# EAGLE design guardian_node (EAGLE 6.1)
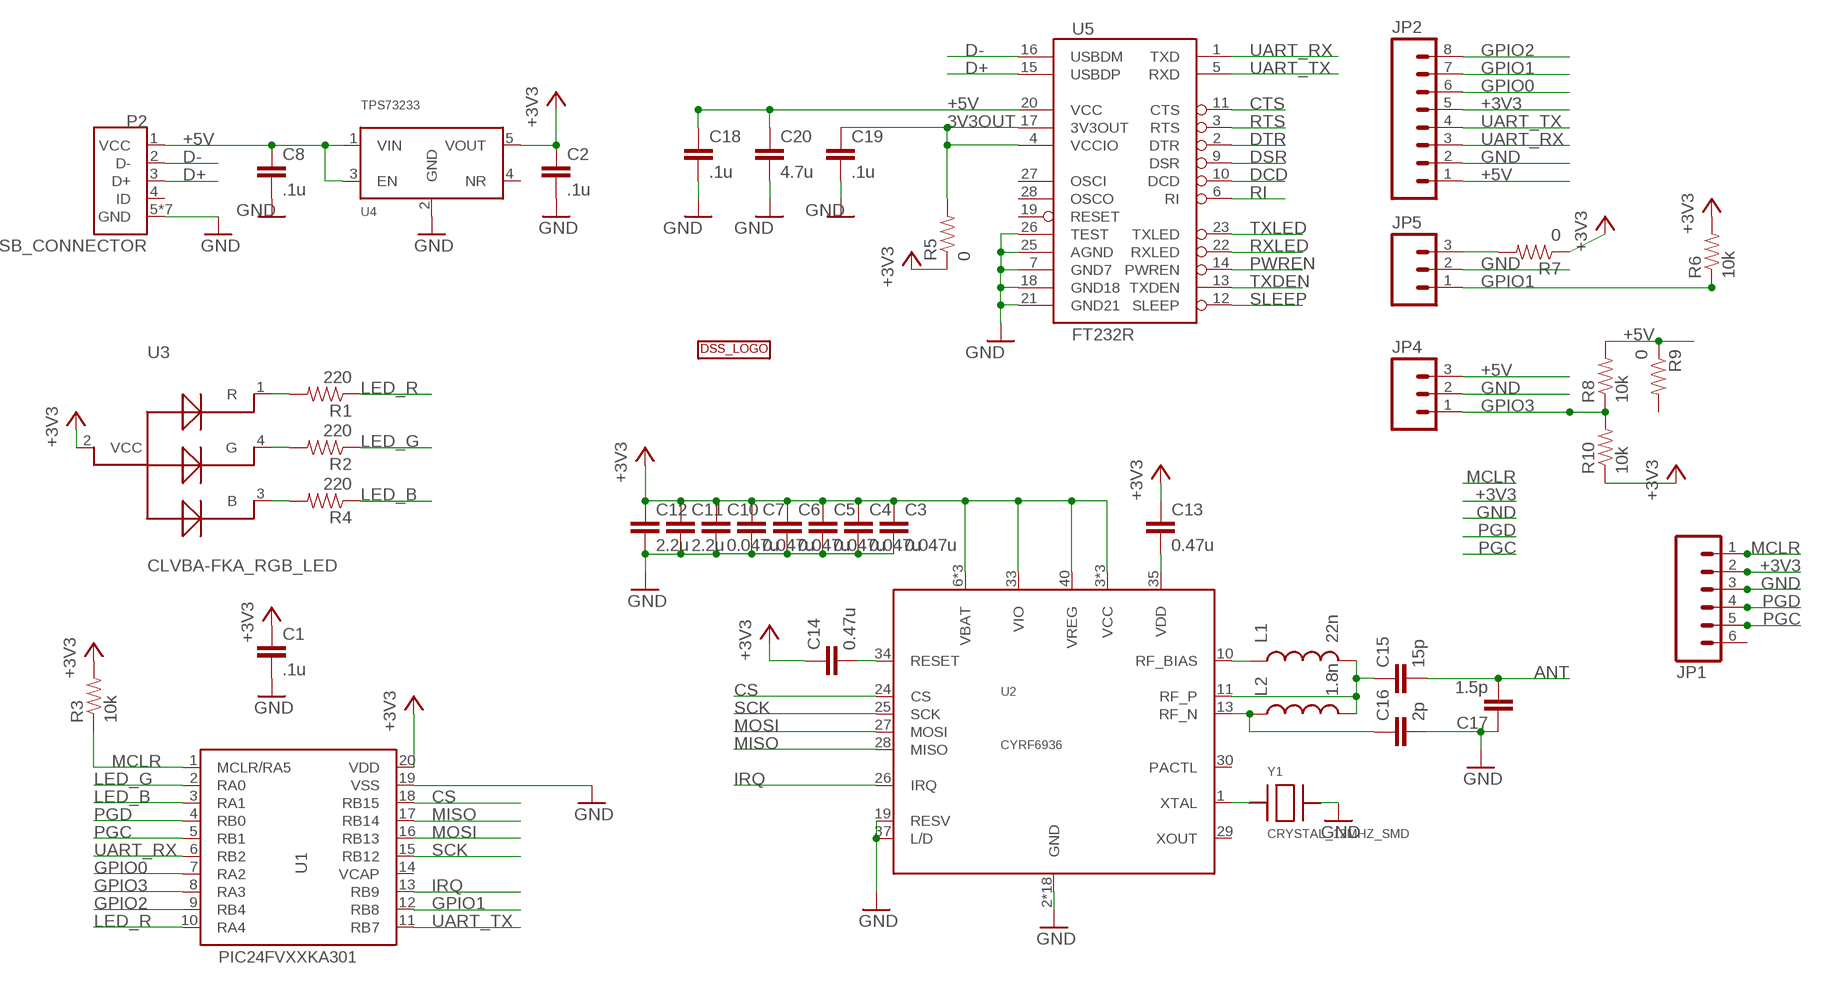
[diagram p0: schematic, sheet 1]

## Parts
C1  .1u  CAP0603-CAP  [0603-CAP]
C2  .1u  CAP0603-CAP  [0603-CAP]
C3  0.047u  CAP0402-CAP  [0402-CAP]
C4  0.047u  CAP0402-CAP  [0402-CAP]
C5  0.047u  CAP0402-CAP  [0402-CAP]
C6  0.047u  CAP0402-CAP  [0402-CAP]
C7  0.047u  CAP0402-CAP  [0402-CAP]
C8  .1u  CAP0603-CAP  [0603-CAP]
C10  0.047u  CAP0402-CAP  [0402-CAP]
C11  2.2u  CAP0402-CAP  [0402-CAP]
C12  2.2u  CAP0402-CAP  [0402-CAP]
C13  0.47u  CAP0402-CAP  [0402-CAP]
C14  0.47u  CAP0402-CAP  [0402-CAP]
C15  15p  CAP0402-CAP  [0402-CAP]
C16  2p  CAP0402-CAP  [0402-CAP]
C17  1.5p  CAP0402-CAP  [0402-CAP]
C18  .1u  CAP0603-CAP  [0603-CAP]
C19  .1u  CAP0603-CAP  [0603-CAP]
C20  4.7u  CAP0603-CAP  [0603-CAP]
JP1  M06SIP  [1X06]
JP2  M081X08  [1X08]
JP4  M03PTH  [1X03]
JP5  M03PTH  [1X03]
L1  22n  INDUCTOR0603  [0603]
L2  1.8n  INDUCTOR0402  [C0402]
P2  USB_CONNECTOR  [USB_MICRO]
R1  220  RESISTOR0402-RES  [0402-RES]
R2  220  RESISTOR0402-RES  [0402-RES]
R3  10k  RESISTOR0603-RES  [0603-RES]
R4  220  RESISTOR0402-RES  [0402-RES]
R5  0  RESISTOR0603-RES  [0603-RES]
R6  10k  RESISTOR0603-RES  [0603-RES]
R7  0  RESISTOR0603-RES  [0603-RES]
R8  10k  RESISTOR0603-RES  [0603-RES]
R9  0  RESISTOR0603-RES  [0603-RES]
R10  10k  RESISTOR0603-RES  [0603-RES]
U1  PIC24FVXXKA301  [SSOP20]
U2  CYRF6936  [QFN40-6X6]
U3  CLVBA-FKA_RGB_LED  [PLCC-4]
U4  TPS73233  [SOT23-5]
U5  FT232R  FT232RLSSOP  [SSOP28DB]
U$1  DSSBOTTOM  [DSS_BOT]
Y1  CRYSTAL_12MHZ_SMD  [SMD-4_5X3.2MM]

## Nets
3V3OUT: C19.1 R5.2 U5.4(VCCIO) U5.17(3V3OUT)
+3V3: C1.1 C2.1 C3.1 C4.1 C5.1 C6.1 C7.1 C10.1 C11.1 C12.1 C13.1 C14.1 JP1.2 JP2.5 R3.2 R5.1 R6.2 R7.1 R10.1 U1.20(VDD) U2.3(VCC) U2.6(VBAT) U2.7(VCC) U2.8(VBAT) U2.16(VCC) U2.33(VIO) U2.38(VBAT) U2.40(VREG) U3.2(VCC) U4.5(VOUT)
+5V: C8.1 C18.1 C20.1 JP2.1 JP4.3 P2.1(VCC) R8.2 R9.1 U4.1(VIN) U4.3(EN) U5.20(VCC)
ANT: C15.2 C17.2
CS: U1.18(RB15) U2.24(CS)
CTS: U5.11(CTS)
D+: P2.3(D+) U5.15(USBDP)
D-: P2.2(D-) U5.16(USBDM)
DCD: U5.10(DCD)
DSR: U5.9(DSR)
DTR: U5.2(DTR)
GND: C1.2 C2.2 C3.2 C4.2 C5.2 C6.2 C7.2 C8.2 C10.2 C11.2 C12.2 C16.2 C17.1 C18.2 C19.2 C20.2 JP1.3 JP2.2 JP4.2 JP5.2 P2.5(GND) P2.GND1(GND) P2.GND2(GND) P2.GND3(GND) P2.GND4(GND) P2.GND5(GND) P2.GND6(GND) U1.19(VSS) U2.2(GND) U2.4(GND) U2.5(GND) U2.9(GND) U2.12(GND) U2.14(GND) U2.15(GND) U2.17(GND) U2.18(GND) U2.19(RESV) U2.20(GND) U2.21(GND) U2.22(GND) U2.23(GND) U2.31(GND) U2.32(GND) U2.36(GND) U2.37(L/D) U2.39(GND) U2.EXP(GND) U4.2(GND) U5.7(GND7) U5.18(GND18) U5.21(GND21) U5.25(AGND) U5.26(TEST) Y1.P$3
GPIO0: JP2.6 U1.7(RA2)
GPIO1: JP2.7 JP5.1 R6.1 U1.12(RB8)
GPIO2: JP2.8 U1.9(RB4)
GPIO3: JP4.1 R8.1 R10.2 U1.8(RA3)
IRQ: U1.13(RB9) U2.26(IRQ)
LED_B: R4.1 U1.3(RA1)
LED_G: R2.1 U1.2(RA0)
LED_R: R1.1 U1.10(RA4)
MCLR: JP1.1 R3.1 U1.1(MCLR/RA5)
MISO: U1.17(RB14) U2.28(MISO)
MOSI: U1.16(RB13) U2.27(MOSI)
N$1: R1.2 U3.1(R)
N$2: R2.2 U3.4(G)
N$3: R4.2 U3.3(B)
N$4: JP5.3 R7.2
N$5: L1.1 U2.10(RF_BIAS)
N$6: C15.1 L1.2 L2.2 U2.11(RF_P)
N$7: C13.2 U2.35(VDD)
N$8: C14.2 U2.34(RESET)
N$9: C16.1 L2.1 U2.13(RF_N)
N$10: U2.1(XTAL) Y1.P$1
PGC: JP1.5 U1.5(RB1)
PGD: JP1.4 U1.4(RB0)
PWREN: U5.14(PWREN)
RI: U5.6(RI)
RTS: U5.3(RTS)
RXLED: U5.22(RXLED)
SCK: U1.15(RB12) U2.25(SCK)
SLEEP: U5.12(SLEEP)
TXDEN: U5.13(TXDEN)
TXLED: U5.23(TXLED)
UART_RX: JP2.3 U1.6(RB2) U5.1(TXD)
UART_TX: JP2.4 U1.11(RB7) U5.5(RXD)
Unconnected: JP1.6 P2.4(ID) R9.2 U1.14(VCAP) U2.29(XOUT) U2.30(PACTL) U4.4(NR) U5.19(RESET) U5.27(OSCI) U5.28(OSCO)

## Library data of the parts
C1-C8 C10-C20 = SparkFun-Passives:CAP: Capacitor
JP1 = SparkFun-Connectors:M06: Header 6 Standard 6-pin 0.1" header. Use with straight break away headers (SKU : PRT-00116), right angle break away headers (PRT-00553), swiss pins (PRT-00743), machine pins (PRT-00117), and female headers (PRT-00115). Molex polarized connector foot print use with SKU : PRT-08094 with associated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
JP2 = SparkFun-Connectors:M08: Header 8 Standard 8-pin 0.1" header. Use with straight break away headers (SKU : PRT-00116), right angle break away headers (PRT-00553), swiss pins (PRT-00743), machine pins (PRT-00117), and female headers (PRT-00115).
JP4 JP5 = SparkFun-Connectors:M03: Header 3 Standard 3-pin 0.1" header. Use with straight break away headers (SKU : PRT-00116), right angle break away headers (PRT-00553), swiss pins (PRT-00743), machine pins (PRT-00117), and female headers (PRT-00115). Molex polarized connector foot print use with SKU : PRT-08232 with associated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
L1 L2 = SparkFun-Passives:INDUCTOR: Inductors
P2 = DSS:USB_CONNECTOR: USB Connector http://www.digikey.com/product-detail/en/10118192-0001LF/609-4613-1-ND/2785378
R1-R10 = SparkFun-Passives:RESISTOR: Resistor
U1 = DSS:PIC24FVXXKA301: PIC24FVXXKA301
U2 = DSS:CYRF6936: Cypress CYRF6936 2.4GHz DSSS radio. All N/C pins and the exposed pad are tied to ground.
U3 = DSS:CLVBA-FKA_RGB_LED
U4 = DSS:TPS73233: TI TPS73233 - fixed output http://www.ti.com/product/tps73233
U5 = SparkFun:FT232RL: USB UART FT232RL 4th Generation USB UART (USB <-> Serial) Controller. Spark Fun Electronics SKU : COM-00650
U$1 = DSS:DSS: DSS LOGO
Y1 = DSS:CRYSTAL_12MHZ_SMD: 12MHz crystal, SMD

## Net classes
2 VCC: width 0.406 mm, clearance 0.381 mm

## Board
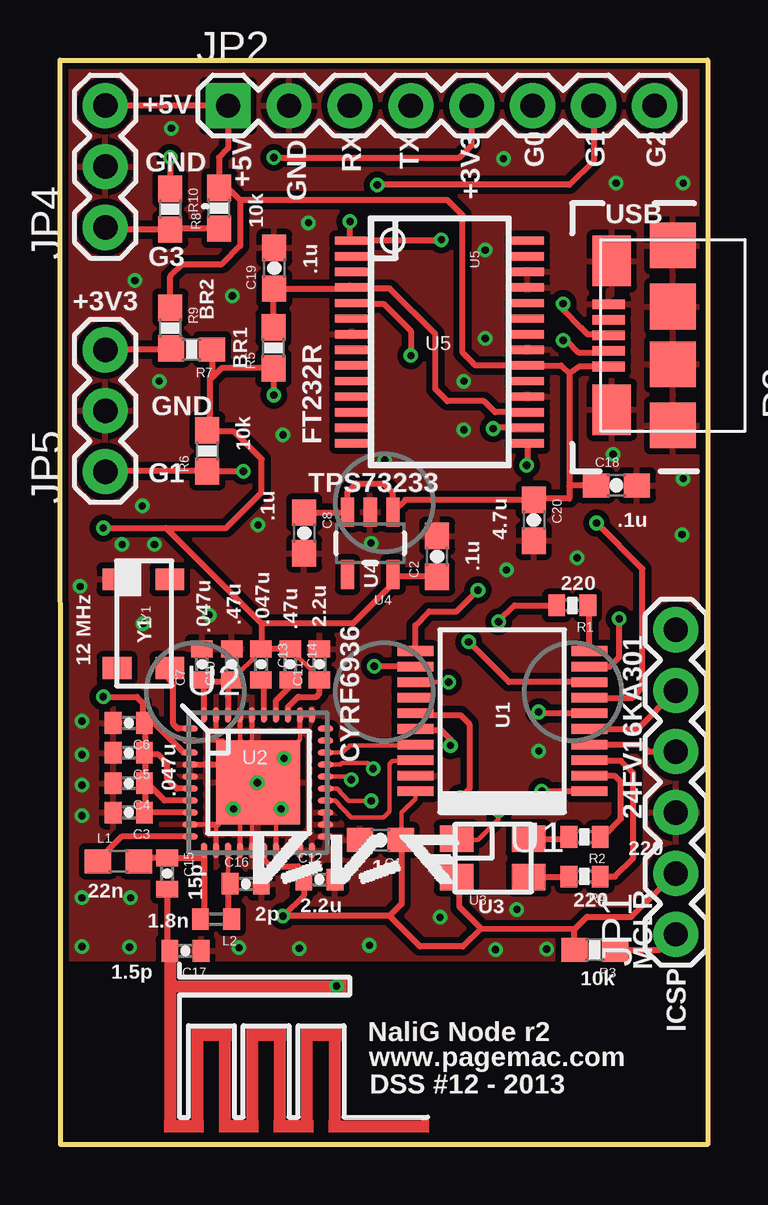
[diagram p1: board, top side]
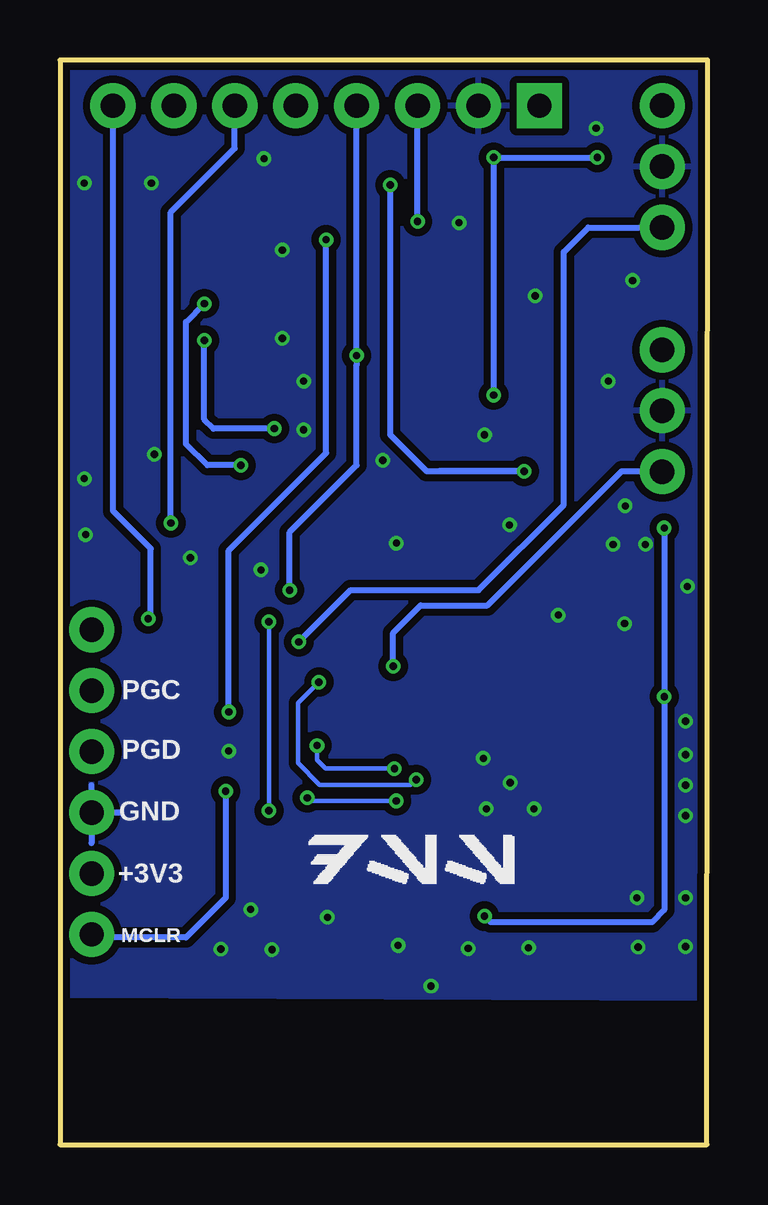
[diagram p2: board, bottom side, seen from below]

Size 27 x 45.21 mm. Coordinates in mm from the lower left corner, seen from the top.
Outline: 0,45.21 27,45.21 27,0 0.03,0 0,45.21
Copper layers (1*16): Top 0.035mm / dielectric 1.5mm / Bottom 0.035mm
Design rules: minimum track width 6mil, minimum drill 12mil, track to track 6mil, track to pad 6mil, pad to pad 6mil, via to via 6mil, smd to smd 0mil, copper to edge 10mil, drill to drill 10mil, minimum pad ring 10mil, minimum via ring 6mil, stop-mask expansion 2mil, vias tented up to drill 100mil, thermal gap 10mil

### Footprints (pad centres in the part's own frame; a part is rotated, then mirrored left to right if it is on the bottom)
0603-CAP = smd 1.1 x 1: 1 -0.85,0; 2 0.85,0
0402-CAP = smd 0.7 x 0.9: 1 -0.65,0; 2 0.65,0
1X06 = drill 1.016 pad 1.88: 1 0,0; 2 2.54,0; 3 5.08,0; 4 7.62,0; 5 10.16,0; 6 12.7,0
1X08 = drill 1.016 pad 1.88 square: 1 0,0 | drill 1.016 pad 1.88: 2 2.54,0; 3 5.08,0; 4 7.62,0; 5 10.16,0; 6 12.7,0; 7 15.24,0; 8 17.78,0
1X03 = drill 1.016 pad 1.88: 1 0,0; 2 2.54,0; 3 5.08,0
0603 = smd 1.1 x 1: 1 -0.85,0; 2 0.85,0
C0402 = smd 0.7 x 0.9: 1 -0.65,0; 2 0.65,0
USB_MICRO = smd 0.4 x 1.35: 1 -1.3,2.675; 2 -0.65,2.675; 3 0,2.675; 4 0.65,2.675; 5 1.3,2.675 | smd 1.9 x 1.9: GND1 -3.75,0; GND2 -1.2,0; GND3 1.2,0; GND4 3.75,0 | smd 2.1 x 1.6: GND5 -3.1,2.55; GND6 3.1,2.55
0402-RES = smd 0.7 x 0.9: 1 -0.65,0; 2 0.65,0
0603-RES = smd 1.1 x 1: 1 -0.85,0; 2 0.85,0
SSOP20 = smd 0.4 x 1.5: 1 -2.925,-3.625; 2 -2.275,-3.625; 3 -1.625,-3.625; 4 -0.975,-3.625; 5 -0.325,-3.625; 6 0.325,-3.625; 7 0.975,-3.625; 8 1.625,-3.625; 9 2.275,-3.625; 10 2.925,-3.625; 11 2.925,3.625; 12 2.275,3.625; 13 1.625,3.625; 14 0.975,3.625; 15 0.325,3.625; 16 -0.325,3.625; 17 -0.975,3.625; 18 -1.625,3.625; 19 -2.275,3.625; 20 -2.925,3.625
QFN40-6X6 = smd 0.65 x 0.25: 1 -2.825,2.25; 2 -2.825,1.75; 3 -2.825,1.25; 4 -2.825,0.75; 5 -2.825,0.25; 6 -2.825,-0.25; 7 -2.825,-0.75; 8 -2.825,-1.25; 9 -2.825,-1.75; 10 -2.825,-2.25; 21 2.825,-2.25; 22 2.825,-1.75; 23 2.825,-1.25; 24 2.825,-0.75; 25 2.825,-0.25; 26 2.825,0.25; 27 2.825,0.75; 28 2.825,1.25; 29 2.825,1.75; 30 2.825,2.25 | smd 0.25 x 0.65: 11 -2.25,-2.825; 12 -1.75,-2.825; 13 -1.25,-2.825; 14 -0.75,-2.825; 15 -0.25,-2.825; 16 0.25,-2.825; 17 0.75,-2.825; 18 1.25,-2.825; 19 1.75,-2.825; 20 2.25,-2.825; 31 2.25,2.825; 32 1.75,2.825; 33 1.25,2.825; 34 0.75,2.825; 35 0.25,2.825; 36 -0.25,2.825; 37 -0.75,2.825; 38 -1.25,2.825; 39 -1.75,2.825; 40 -2.25,2.825 | smd 3.5 x 3.5: EXP 0,0
PLCC-4 = smd 1.4 x 1.1: 1 -1.524,0.812; 2 -1.524,-0.788; 3 1.476,-0.788; 4 1.476,0.812
SOT23-5 = smd 0.55 x 1.2: 1 -0.95,-1.3; 2 0,-1.3; 3 0.95,-1.3; 4 0.95,1.3; 5 -0.95,1.3
SSOP28DB = smd 0.348 x 1.397: 1 -4.225,-3.656; 2 -3.575,-3.656; 3 -2.925,-3.656; 4 -2.275,-3.656; 5 -1.625,-3.656; 6 -0.975,-3.656; 7 -0.325,-3.656; 8 0.325,-3.656; 9 0.975,-3.656; 10 1.625,-3.656; 11 2.275,-3.656; 12 2.925,-3.656; 13 3.575,-3.656; 14 4.225,-3.656; 15 4.225,3.656; 16 3.575,3.656; 17 2.925,3.656; 18 2.275,3.656; 19 1.625,3.656; 20 0.975,3.656; 21 0.325,3.656; 22 -0.325,3.656; 23 -0.975,3.656; 24 -1.625,3.656; 25 -2.275,3.656; 26 -2.925,3.656; 27 -3.575,3.656; 28 -4.225,3.656
SMD-4_5X3.2MM = smd 0.9 x 1.2: P$1 1.9,1.1; P$2 1.9,-1.1; P$3 -1.8,-1.1; P$4 -1.8,1.1

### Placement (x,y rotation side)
C1  13.36,12.7 180 top
C2  15.73,24.52 90 top
C3  2.87,13.84 180 top
C4  2.87,15.06 180 top
C5  2.87,16.33 180 top
C6  2.87,17.58 180 top
C7  5.92,20.02 90 top
C8  10.18,25.5 270 top
C10  7.16,20.02 90 top
C11  10.82,20.02 90 top
C12  10.82,11.05 0 top
C13  8.38,20.02 270 top
C14  9.6,20.02 270 top
C15  4.47,11.3 270 top
C16  7.75,10.87 0 top
C17  5.23,8.08 180 top
C18  23.2,27.48 0 top
C19  8.94,36.53 90 top
C20  19.76,26.03 270 top
JP1  25.68,8.76 90 top
JP2  7.01,43.31 0 top
JP4  1.89,38.23 90 top
JP5  1.89,28.05 90 top
L1  2.44,11.81 0 top
L2  6.5,9.4 180 top
P2  25.55,33.73 90 top
R1  21.36,22.48 180 top
R2  21.87,12.83 180 top
R3  22.3,8.13 180 top
R4  21.87,11.18 180 top
R5  8.9,33.21 90 top
R6  6.15,28.92 90 top
R7  5.49,33.15 180 top
R8  6.64,39.03 90 top
R9  4.6,34.04 270 top
R10  4.6,38.99 270 top
U1  18.44,17.65 90 top
U2  8.25,15.09 0 top
U3  18.06,11.94 0 top
U4  12.94,25.06 180 top
U5  15.83,33.45 270 top
U$1  7.9,10.67 0 top
Y1  3.48,21.77 270 top

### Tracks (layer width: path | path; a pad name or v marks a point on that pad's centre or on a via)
3V3OUT
  Top 0.254: U5.17 18.14,30.53 17.68,30.99 16.15,30.99 15.65,31.5 15.65,33.78 13.74,35.69 12.22,35.69 | 12.22,35.69 12.09,35.81 | R5.2 8.9,35.65 C19.1 12.12,35.68 U5.4 12.21,35.69 12.22,35.69
+3V3  (via drill 0.3)
  Top 0.178: U2.33 9.52,17.91 9.55,17.88 | 10.82,19.45 C14.1 | 8.38,20.58 C10.1 | U1.20 14.82,14.41 14.25,13.84 14.25,12.74 C1.1 | 10.19,11.3 C12.1
  Top 0.254: 3.58,13.84 U2.8 3.59,13.84 3.58,13.84 | U2.7 4.36,14.34 3.71,14.99 3.6,14.99 C4.1 3.57,15.11 3.58,15.11 | 3.45,16.39 C5.1 | U2.38 7.01,18.67 7.04,19.46 C10.1 7.1,19.3 5.99,19.3 6.01,19.29 U2.40 6.01,19.17 5.87,19.3 5.92,19.36 C7.1 | U2.16 8.51,11.89 8.79,11.61 9.93,11.61 10.19,11.3 | 10.82,19.45 C11.1 10.82,18.8 10.69,18.67 9.93,18.67 9.51,18.24 U2.33 | C14.1 C13.1 | C13.1 8.38,20.58 | 8.41,20.64 8.41,21.72 8.42,21.7 8.43,21.7 | v1.8,18.67 3.2,18.67 3.45,18.41 3.45,17.64 C6.1 3.57,17.53 3.58,17.53 | U2.6 4.87,14.84 4.47,15.24 4.47,15.88 4.09,16.26 3.45,16.26 3.45,16.27 C5.1 | U2.3 5.15,16.34 3.96,17.53 3.58,17.53 | 3.45,13.72 3.58,13.84 | C3.1 3.58,13.84 | 3.58,13.84 3.58,15.11 | 3.58,15.11 3.58,16.38 | 3.58,16.38 3.58,17.53 | C5.1 3.53,16.33 3.58,16.38 | 8.41,20.57 8.41,20.64 | 8.41,20.64 C13.1 | 16.43,11.05 U3.2 | R3.2 21.45,8.98 | 21.45,8.98 21.97,9.5 23.83,9.5 JP1.2 | 21.45,8.98 17.57,9 17.55,9.02 | 17.55,9.02 16.66,9.91 16.66,11.02 U3.2 | 16.51,11.18 U3.2 | 14.25,12.74 14.25,10.03 13.74,9.53 | 13.74,9.53 v9.3,9.53 10.17,10.4 C12.1 | 17.55,9.02 16.79,8.26 15.01,8.26 13.74,9.53 | v1.8,25.7 4.42,25.7 | 4.42,25.7 8.43,21.7 | C2.1 13.98,23.67 U4.5 13.89,23.39 12.22,21.72 8.44,21.72 8.43,21.7 | 6.25,31.88 6.25,32 6.34,32.09 R7.1 | 6.25,31.88 6.25,29.84 6.17,29.77 R6.2 6.2,29.77 6.25,29.72 7.26,29.72 8.41,28.57 8.41,27.18 6.93,25.7 4.42,25.7 | 6.25,31.88 6.73,32.36 R5.1 8.9,31.25 v8.92,31.24 | v8.92,41.15 16.66,41.15 17.17,41.66 JP2.5 | v4.6,41.15 R10.1
  Bottom 0.254: v1.8,25.7 v1.8,18.67 1.8,9.78 2.31,9.27 9.04,9.27 v9.3,9.53 | v8.92,31.24 v8.92,41.15 v4.6,41.15
+5V
  Top 0.254: C8.1 11.97,26.35 U4.3 11.99,27.2 12.34,27.56 13.49,27.56 13.87,27.18 13.87,26.42 | 13.87,26.42 13.87,26.38 U4.1 14.4,26.88 C20.1 19.81,26.92 21.23,26.92 21.23,27.43 | P2.1 21.66,32.43 21.23,32.13 | 21.23,32.13 21.23,27.43 | 14,26.29 13.87,26.42 | 21.23,32.13 20.89,32.48 U5.20 17.33,32.48 16.79,33.02 16.79,38.73 16.15,39.37 7.52,39.37 | JP4.3 JP2.1 7.01,41.53 6.63,41.15 R8.2 7.01,39.88 7.52,39.37 | C18.1 21.28,27.48 21.23,27.43 | R9.1 4.6,36.2 5.11,36.7 6.76,36.7 7.52,37.47 7.52,39.37
ANT
  Top 0.254: C15.2 4.47,8.29 C17.2
CS
  Top 0.178: U2.24 11.47,14.34 12.14,13.64 13.49,13.64 13.74,13.89 13.74,15.88 13.87,16 14.79,16
  Top 0.254: 14.79,16 U1.18
D+  (via drill 0.3)
  Top 0.254: U5.15 19.48,28.35 v19.46,28.32 | v20.98,35.05 20.98,34.8 21.74,34.04 22,33.78 22.83,33.78 P2.3
  Bottom 0.254: v19.46,28.32 20.85,28.32 21.74,29.21 21.74,34.29 v20.98,35.05
D-  (via drill 0.3)
  Top 0.254: U5.16 18.09,29.88 v18.06,29.84 | v20.98,33.53 21.11,33.53 21.62,33.02 22.82,33.02 P2.2
  Bottom 0.254: v18.06,29.84 20.6,29.84 20.98,30.23 v20.98,33.53
GND  (via drill 0.3)
  Top 0.178: U2.9 6.12,13.34 | U2.12 6.51,13.26 6.86,13.61 v7.24,13.99 | U2.17 9.01,13.51 | 9.01,13.51 9.01,13.91 v9.22,13.99 | U2.15 8.01,13.41 8.08,13.49 8.08,13.41 8.9,13.41 9.01,13.51 | U2.14 7.51,13.73 | 6.97,15.84 7.47,15.82 | U2.2 6.55,16.84 | 6.55,16.84 6.78,16.84 7.04,16.59 7.04,16.26 7.47,15.82 | U2.39 6.51,16.89 6.55,16.84 | U2.37 7.51,16.88 7.65,16.74 7.65,16.48 7.26,16.1 | U2.36 8.01,16.87 7.26,16.13 7.47,15.82 | U2.32 10.01,16.89 v9.35,16.1 | 10.03,17.91 U2.31 | U2.31 | U2.31 | U2.23 U2.22
  Top 0.254: U2.4 6.97,15.84 7.26,16.13 | 6.12,13.34 6.58,13.34 6.86,13.61
  Top 0.508: 4.6,8.26 4.6,6.6 | 4.6,6.6 4.6,0.76 5.74,0.76 5.74,4.57 6.88,4.57 6.88,0.76 | 4.6,6.6 v11.53,6.6 11.68,6.6
  Bottom 0.254: JP1.3 24.46,13.84 | JP1.3 25.68,14.99 | JP1.3 25.68,12.57
  other vias: 3.94,25.02 9.98,8.18 6.22,22.07 15.85,9.47 0.91,17.65 7.47,8.2 0.91,8.26 0.91,10.29 8.23,15.09 2.9,8.23 25.93,25.43 0.91,16.26 0.91,14.99 0.91,13.72 2.95,10.29 18.16,8.13 20.29,8.15 0.84,23.27 3.45,21.72 21.56,24.46 2.59,25.02 19.05,9.8 3.43,26.62 4.14,31.83 12.97,25.07 9.3,29.59 8.25,25.83 18.62,23.95 16.84,29.79 23.19,40.08 13.54,28.52 25.98,40.08 25.98,27.76 19.96,16.41 12.9,8.31 17.73,37.29 3.12,36.02 7.19,35.38 4.65,42.37 23.06,28.78 18.49,41.1 10.36,38.43 16.84,31.83 17.73,33.6
  pour Top (isolate 0.254): -0.36,45.71 27.22,45.85 27.09,7.72 0.15,7.7
  pour Bottom (isolate 0.305): 0.03,6.07 26.95,6.2 27.2,45.85 -0.33,45.67
GPIO0  (via drill 0.3)
  Top 0.254: U1.7 23.86,18.63 24.28,19.05 24.28,24 v22.38,25.91
  Bottom 0.254: v22.38,25.91 22.38,38.86 19.71,41.53 JP2.6
GPIO1  (via drill 0.3)
  Top 0.254: U1.12 13.12,19.93 v13.11,19.94 | JP5.1 1.91,28.07 R6.1 v7.65,28.07 | JP2.7 22.25,41.02 21.23,40.01 v13.23,40.01 | v7.65,28.07
  Bottom 0.254: v13.11,19.94 13.11,21.34 11.96,22.48 9.17,22.48 3.58,28.07 1.93,28.07 1.91,28.07 JP5.1 | v13.23,40.01 13.23,29.59 11.71,28.07 11.2,28.07 | 11.2,28.07 v7.65,28.07 11.2,28.07
GPIO2  (via drill 0.3)
  Top 0.254: U1.9 22.93,19.93 23.32,20.32 v23.32,21.92
  Bottom 0.254: v23.32,21.92 23.22,21.97 23.22,24.84 24.79,26.42 JP2.8
GPIO3  (via drill 0.3)
  Top 0.254: U1.8 18.72,19.28 v17.04,20.95 | R8.1 4.64,38.18 R10.2 2.02,38.14 1.93,38.23 JP4.1
  Bottom 0.254: v17.04,20.95 14.88,23.11 9.55,23.11 5.99,26.67 5.99,37.21 4.98,38.23 JP4.1
IRQ  (via drill 0.3)
  Top 0.178: U2.26 12.02,15.34 v12.14,15.21 | U1.13 v16.2,19.28 v16.21,19.28
  Bottom 0.178: v12.14,15.21 12.4,14.99 16.18,14.99 17.07,15.9 17.07,18.41 v16.21,19.28
LED_B
  Top 0.254: R4.1 23.14,11.18 23.9,11.94 23.9,15.49 23.39,16 22.09,16 U1.3
LED_G
  Top 0.254: R2.1 22.63,12.83 23.39,13.59 23.39,15.11 23.14,15.37 22.08,15.37 U1.2
LED_R
  Top 0.254: U1.10 22.07,22.43 R1.1
MCLR  (via drill 0.3)
  Top 0.254: U1.1 v20.1,14.73 v20.09,14.73 | R3.1 25.02,8.13 JP1.1
  Bottom 0.254: v20.09,14.73 20.09,10.29 21.74,8.64 25.55,8.64 JP1.1
MISO
  Top 0.178: U2.28 11.79,16.34 12.09,16.64 14.77,16.64
  Top 0.254: 14.77,16.64 U1.17
MOSI  (via drill 0.3)
  Top 0.178: U2.27 11.7,15.84 11.76,15.9 12.83,15.9 v13.06,15.67
  Top 0.254: U1.16 14.87,17.27 14.88,17.27 15.9,17.27 16.28,16.89 v16.28,16.64
  Bottom 0.178: v13.06,15.67 15.93,15.67 16.28,16.03 v16.28,16.64
N$1  (via drill 0.3)
  Top 0.178: v18.29,13.92 18.29,13.56 17.42,12.7 16.59,12.7 U3.1
  Top 0.254: R1.2 18.95,22.48 18.29,21.82 v18.29,21.79
  Bottom 0.178: v18.29,21.79 v18.29,13.92
N$2
  Top 0.254: U3.4 21.4,12.75 R2.2
N$3
  Top 0.254: U3.3 21.45,11.15 R4.2
N$4
  Top 0.254: R7.2 2.03,33.15 | 2.03,33.15 1.91,33.15 JP5.3 | 4.76,33.15 2.03,33.15
N$5
  Top 0.254: U2.10 2.58,12.84 1.42,11.68 1.42,11.72 L1.1
N$6
  Top 0.254: U2.11 6.01,11.05 | 6.01,11.05 6.01,9.54 5.87,9.4 L2.2 | 6.01,11.05 5.99,11.95 C15.1 3.18,11.95 L1.2
N$7
  Top 0.254: U2.35 8.51,19.24 C13.2
N$8
  Top 0.254: U2.34 9.01,18.5 9.55,19.05 9.55,19.31 C14.2
N$9
  Top 0.178: U2.13 7,10.48
  Top 0.254: 7,10.48 C16.1 7.04,10.49 | L2.1 7.04,9.53 7.04,10.49 | 7.04,10.49 7.04,10.54 | 7.04,10.54 7.04,10.49 | 7.04,10.49 7.04,10.54
N$10
  Top 0.254: U2.1 4.91,17.34 4.72,17.53 4.72,19.18 4.34,19.68 4.6,19.81 4.58,19.92 Y1.P$1
N$11
  Top 0.508: 6.88,0.76 8.03,0.76 8.03,4.57 9.17,4.57 9.17,0.76
N$12
  Top 0.508: 9.17,0.76 10.31,0.76 10.31,4.57 11.46,4.57 11.46,0.76 15.14,0.76
PGC
  Top 0.254: U1.5 24.08,17.33 JP1.5
PGD
  Top 0.254: U1.4 24.24,16.68 24.54,16.38 JP1.4
SCK  (via drill 0.3)
  Top 0.178: U2.25 11.55,14.84 12.04,14.33 v12.98,14.33
  Top 0.254: U1.15 14.89,17.91 16.69,17.91 17.07,17.53 17.07,14.83 v16.69,14.45
  Bottom 0.178: v12.98,14.33 16.51,14.33 16.66,14.48 v16.69,14.45
UART_RX  (via drill 0.3)
  Top 0.254: U1.6 19.96,17.98 v19.96,18.03 | v15.9,37.72 15.61,37.68 U5.1 12.09,37.76 v12.09,38.48
  Bottom 0.254: v19.96,18.03 19.96,24.77 15.9,28.83 v15.9,37.72 | 12.09,43.43 JP2.3 v12.09,38.48
UART_TX  (via drill 0.3)
  Top 0.254: U1.11 14.82,21.65 15.39,22.23 16.54,22.23 v17.42,23.11 | U5.5 12.2,35.05 13.49,35.05 14.63,33.91 v14.63,32.89
  Bottom 0.254: v17.42,23.11 17.42,25.53 14.63,28.32 14.63,32.51 v14.63,32.89 JP2.4
(copper drawn outside any net)
  shapes: Top area x9

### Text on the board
tDocu: B0 | B3 | B4 | B2 | B1
_tsilk: +5V | +5V | GND | RX | TX | +3V3 | G0 | G1 | G2 | GND | 10k | USB | G3 | .1u | +3V3 | BR2 | FT232R | U5 | BR1 | GND | 10k | G1 | TPS73233 | 4.7u | .1u | .1u | .1u | .047u | 220 | 12 MHz | .47u | U4 | Y1 | 2.2u | .047u | .47u | 24FV16KA301 | U1 | .047u | U2 | CYRF6936 | 220 | 15p | .1u | 220 | 22n | 1.8n | 2.2u | U3 | 2p | 1.5p | 10k | MCLR | ICSP | NaliG Node r2 | www.pagemac.com | DSS #12 - 2013
_bsilk: PGC | PGD | GND | +3V3 | MCLR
